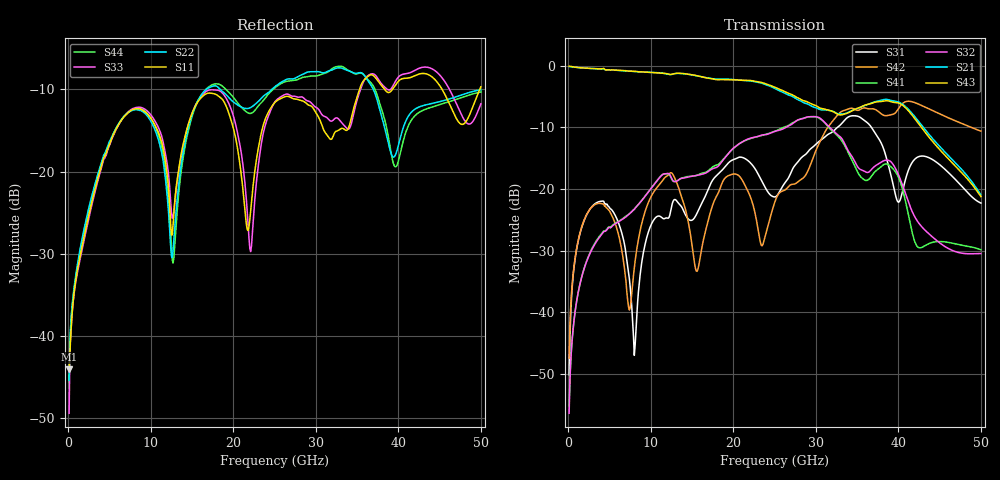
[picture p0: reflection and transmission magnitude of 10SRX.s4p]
! DAC39RF10ACK
! 256-pin FCBGA package
! Texas Instruments 8/20/2022
! Single-ended  S-parameters
! PORT#  PORT_NAME  NET_NAME
! PORT1:  xSRXN.DIEBUMP  xSRXN
! PORT2:  xSRXN.BGA  xSRXN
! PORT3:  xSRXP.DIEBUMP  xSRXP
! PORT4:  xSRXP.BGA  xSRXP
! Touchstone Ver. 1.0
! Number of ports is 4
# Hz	S	MA	R	50.000000
! SCATTERING PARAMETERS  :
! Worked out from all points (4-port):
!   500 points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, 100 MHz to 50 GHz, reference 50 ohm
!   strongest paths, dB at 100 MHz, 12.6 GHz, 25.1 GHz, 37.6 GHz, 50 GHz:
!     S43: 0.0, -1.3, -3.5, -5.8, -21.2
!     S21: -0.1, -1.4, -3.7, -5.7, -20.9
!     S32: -56.5, -18.5, -10.6, -15.9, -30.5
!     S41: -55.2, -18.6, -10.6, -16.7, -29.9
!     S42: -47.5, -17.5, -21.8, -7.4, -10.6
!     S31: -50.2, -22.4, -21.3, -11.8, -22.3
!   lowest |S11| = -44.1 dB at 100 MHz (marker M1), VSWR 1.01, Z = 50.6 + j0.247 ohm
!   |S11| at or under -10 dB: start of sweep to 35.29 GHz; 38.33 GHz to 39.29 GHz (955 MHz wide, 2.46 % of centre); 45.3 GHz to 49.86 GHz (4.557 GHz wide, 9.58 % of centre)
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1e8  0.006263 23.0  0.9927 -2.7  0.004081 81.6  0.001364 -100.2
     0.9889 -2.6  0.005373 37.1  0.00135 -88.2  0.004232 81.6
     0.003093 68.2  0.001503 -102.5  0.003385 50.0  0.9938 -2.7
     0.001728 -96.7  0.004223 81.3  0.9959 -2.7  0.00525 36.7
3.7e9  0.09536 19.4  0.9457 -83.9  0.07881 0.4  0.04015 174.6
       0.9468 -83.9  0.101 -24.6  0.04024 175.1  0.07644 7.8
       0.07879 0.4  0.0399 175.0  0.09257 19.3  0.9471 -83.2
       0.04061 174.9  0.07641 7.7  0.9477 -83.0  0.09807 -23.7
7.9e9  0.2396 -67.7  0.9 -177.2  0.006706 -149.3  0.06751 90.9
       0.9028 -177.2  0.2369 -108.4  0.06785 91.6  0.02029 143.8
       0.006351 -147.8  0.06776 91.6  0.2429 -66.5  0.8987 -175.7
       0.06753 90.8  0.01985 142.6  0.9053 -175.6  0.2398 -107.0
1.27e10  0.04772 -78.7  0.8598 77.6  0.07867 -17.8  0.1155 -29.6
         0.8595 77.6  0.03322 20.3  0.1157 -29.1  0.1315 13.6
         0.07949 -17.8  0.1165 -29.1  0.05295 -95.0  0.8607 80.1
         0.1156 -29.4  0.1306 14.2  0.8598 80.1  0.02776 43.5
1.57e10  0.2658 -89.0  0.8278 8.1  0.06443 161.9  0.1301 -86.8
         0.8281 8.1  0.2701 -78.1  0.1289 -86.1  0.02314 34.4
         0.06559 161.8  0.1293 -86.0  0.2692 -86.4  0.827 10.9
         0.1303 -86.7  0.02216 37.3  0.8304 10.9  0.2688 -75.5
2.35e10  0.1814 -42.8  0.7213 -169.2  0.1147 -121.2  0.2715 93.2
         0.7225 -169.3  0.2831 -122.8  0.2738 95.9  0.03466 12.7
         0.1144 -121.4  0.2747 95.8  0.1589 -39.5  0.7287 -163.9
         0.2729 92.9  0.03457 16.6  0.732 -163.9  0.2659 -122.2
5e10  0.328 -87.4  0.1045 1.8  0.07708 -105.1  0.0239 -126.6
      0.08971 -3.0  0.3144 -140.0  0.03464 -130.6  0.2987 -28.3
      0.07684 -104.9  0.02987 -136.2  0.2586 -92.8  0.1096 15.6
      0.03207 -122.8  0.2953 -28.2  0.0869 10.8  0.305 -138.6
